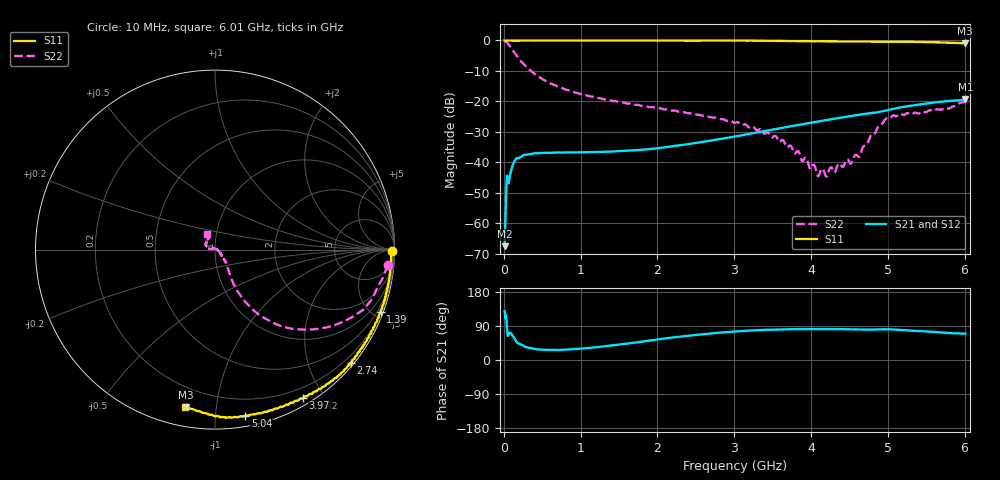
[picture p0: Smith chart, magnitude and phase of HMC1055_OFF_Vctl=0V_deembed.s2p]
! Device:	HMC1055
! Description:	GaAs MMIC SPST Switch
! Package:	LP2 8 pin 2x2 mm QFN Plastic Package
! Frequency:	0.5 -  4 GHz
! Ports:
! RF1 = Port 1
! RF2 = Port 2
! State: OFF
! Supply Votage: Vdd = 3 V
! ControlVoltage: Vctl = 0 V
! Data:	Data was collected using a calibrated network analyzer with AFR software.
!	Fixtures were calculated using AFR and fixturing was applied to collect
!	this Deembedded  S Parameter data of HMC1055.
!  The reference plane is the edge of the package pin.
! Note:	Analog Devices supplies this data as a sample of measured data at the package pin
!	for this product.  Your particular data for this product may vary.
!	Data was taken at 25 degrees C.
!	Analog Devices reserves the right to change this data at anytime.
# Hz S  dB  R 50
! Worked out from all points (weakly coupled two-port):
!   601 points, 10 MHz to 6.01 GHz, reference 50 ohm
!   highest |S21| = -19.43 dB at 6.01 GHz (marker M1); lowest = -67.5 dB at 10 MHz (marker M2)
!   lowest |S11| = -1.0 dB at 6 GHz (marker M3), VSWR 17.31, Z = 4.88 - j41.4 ohm
!   |S11| at or under -10 dB: nowhere
!   |S22| runs from -44.7 to -0.3 dB; largest |S21 - S12| = 0.00071
!   S11 on the Smith chart (normalised r, x): 10 MHz: open; 1.39 GHz: 0.24, -5.51; 2.74 GHz: 0.07, -2.76; 3.97 GHz: 0.08, -1.75; 5.04 GHz: 0.07, -1.20; 6.01 GHz: 0.10, -0.82
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1e7  -0.11 -0.4  -67.50 128.9  -68.47 103.4  -0.31 -5.2
6e7  -0.14 -1.1  -46.91 65.0  -46.86 66.8  -1.35 -25.8
1.5e8  -0.15 -2.4  -39.25 53.0  -39.23 52.4  -4.51 -47.1
2.4e8  -0.15 -3.6  -37.94 39.5  -37.88 39.5  -7.37 -56.4
3.8e8  -0.16 -5.7  -37.19 30.3  -37.07 29.7  -10.65 -60.9
1.01e9  -0.13 -14.8  -36.75 30.0  -36.73 30.0  -17.72 -56.2
1.39e9  -0.13 -20.5  -36.52 37.9  -36.49 37.9  -19.78 -51.6
2.01e9  -0.10 -29.6  -35.39 54.4  -35.36 54.4  -22.33 -48.3
2.74e9  -0.14 -39.8  -32.73 70.8  -32.70 70.7  -25.35 -44.2
3.01e9  -0.13 -43.6  -31.56 75.4  -31.51 75.2  -27.07 -41.7
3.54e9  -0.24 -51.8  -29.14 80.6  -29.09 80.3  -31.40 -25.2
3.97e9  -0.34 -59.3  -27.19 81.8  -27.17 81.5  -41.05 19.7
4.01e9  -0.35 -59.8  -27.01 81.9  -26.99 81.6  -41.49 12.5
4.09e9  -0.36 -61.2  -26.65 81.8  -26.63 81.6  -44.57 41.2
4.15e9  -0.40 -62.5  -26.40 81.8  -26.38 81.5  -42.16 59.1
4.2e9  -0.38 -63.2  -26.17 81.7  -26.16 81.5  -44.74 72.8
4.52e9  -0.47 -69.2  -24.84 81.1  -24.82 80.9  -40.47 132.2
5.01e9  -0.53 -79.0  -22.86 81.0  -22.83 80.8  -25.77 162.0
5.04e9  -0.53 -79.7  -22.70 80.9  -22.67 80.6  -25.30 156.6
5.79e9  -0.85 -95.0  -19.93 71.2  -19.90 71.0  -22.47 117.9
6e9  -1.00 -100.4  -19.47 69.5  -19.43 69.3  -20.30 116.8
6.01e9  -1.00 -100.7  -19.43 69.4  -19.40 69.2  -20.20 116.4
